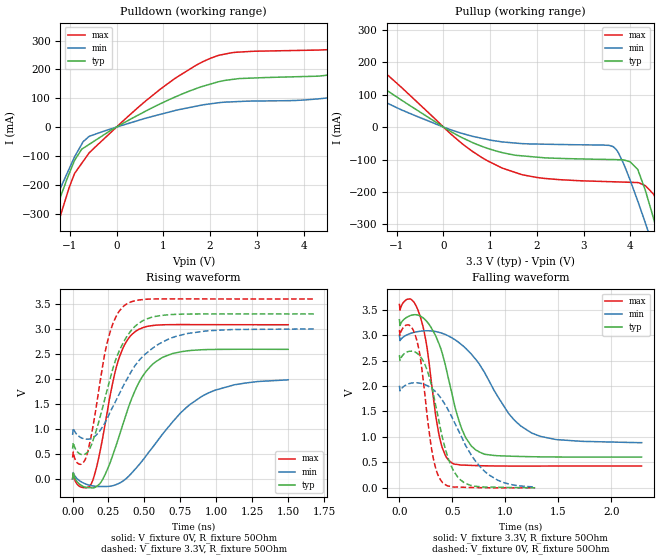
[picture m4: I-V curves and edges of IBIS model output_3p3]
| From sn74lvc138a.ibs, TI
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|   output_3p3 Model
[Model]   output_3p3
Model_type   Output
Polarity   Non-Inverting
Vmeas = 1.65
Vref = 1.65
Cref = 2pF
Rref = 50
|   typ   min   max
|   (nom PVT)   (fast PVT)   (slow PVT)
|C_comp from frequency sweep method (F=5MHz)
|C_comp   6.810e-12   6.693e-12   8.623e-12
|ON state : BUFFER OUTPUT TURNED HIGH
|C_comp   6.810e-12   6.693e-12   8.623e-12
|OFF state: BUFFER OUTPUT TURNED LOW
|C_comp   6.538e-12   6.289e-12   6.590e-12
|C_comp from LC tank measurement(L=1nH)
|Resonant Frequency(Hz)   2.010e+09   2.070e+09   1.960e+09
C_comp   6.276e-12   5.917e-12   6.600e-12
|ON state : BUFFER OUTPUT TURNED HIGH
|Resonant Frequency(Hz)   2.010e+09   2.070e+09   1.960e+09
|C_comp   6.276e-12   5.917e-12   6.600e-12
|OFF state: BUFFER OUTPUT TURNED LOW
|Resonant Frequency(Hz)   2.260e+09   2.290e+09   2.140e+09
|C_comp   4.964e-12   4.835e-12   5.537e-12
| Where nom  PVT is Nominal Process, 3.3V, 27C
|   Fast PVT is Strong Process,  3.6V, -40C
|   Slow PVT is Weak Process,   3V, 125C
[Voltage Range]   3.3   3   3.6
|Ambient Temperature   25   85   -40
|Junction Temperature
[Temperature Range]   27   125   -40
[Pullup Reference]   3.3   3   3.6
[Pulldown Reference]   0   0   0
[Power Clamp Reference]   3.3   3   3.6
[GND Clamp Reference]   0   0   0
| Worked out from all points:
|   slope of the pulldown table from 0 to 0.495 V, typ, clamps not added: 11.2 ohm
|   slope of the pullup table from 0 to 0.495 V, typ, clamps not added: 12.6 ohm
|   falling waveform, V_fixture 3.3V, R_fixture 50Ohm: 20-80 % time 206ps typ, 396ps min, 129ps max; typ from 3.3 V to 0.604 V
|   rising waveform, V_fixture 0V, R_fixture 50Ohm: 20-80 % time 207ps typ, 371ps min, 134ps max; typ from 0 V to 2.59 V
|   rising waveform, V_fixture 3.3V, R_fixture 50Ohm: 20-80 % time 177ps typ, 283ps min, 121ps max; typ from 0.605 V to 3.3 V
|   falling waveform, V_fixture 0V, R_fixture 50Ohm: 20-80 % time 177ps typ, 323ps min, 114ps max; typ from 2.61 V to 0.001 V
[Pulldown]
|   Voltage   I(typ)   I(min)   I(max)
-3.3V     -1.387A    -1.148A    -1.732A
-1.689V   -475.7mA   -405.4mA   -579.7mA
-1.308V   -291.1mA   -250.7mA   -366.8mA
-897.6mV  -115.5mA   -103mA     -161.1mA
-745.8mV  -76.85mA   -59.62mA   -126.1mA
-591mV    -60.58mA   -32.91mA   -90.57mA
939.6mV   81.03mA    44.25mA    131.8mA
2.012V    149.3mA    80.72mA    239mA
2.542V    166.6mA    88.11mA    259.4mA
4.95V     191.9mA    111mA      279.8mA
6V        240.9mA    146mA      341mA
6.6V      273.7mA    165.9mA    382.6mA
[Pullup]
|   Voltage   I(typ)   I(min)   I(max)
-3.3V     312.5mA    216.6mA    431.8mA
-3V       283.8mA    196.2mA    393.1mA
-897.6mV  83.18mA    52.99mA    122.3mA
392.4mV   -32.21mA   -19.31mA   -50.19mA
1.246V    -78.24mA   -45.48mA   -125.5mA
3.63V     -100.1mA   -60.21mA   -168.6mA
4.158V    -130.7mA   -228.1mA   -171.1mA
4.331V    -200.3mA   -299.9mA   -182mA
4.468V    -267.5mA   -358.7mA   -202.7mA
4.687V    -384.2mA   -456.2mA   -293.7mA
4.848V    -470.4mA   -528.2mA   -403mA
6.6V      -1.488A    -1.345A    -1.68A
[Ramp]
R_load = 50
|   typ   min   max
dV/dt_r   1.55471/2.06702e-10   1.19608/3.73506e-10   1.85065/1.33968e-10
dV/dt_f   1.61692/2.05325e-10   1.27163/3.97542e-10   1.90305/1.28863e-10
[Falling Waveform]
V_fixture = 3.3V
V_fixture_min = 3V
V_fixture_max = 3.6V
R_fixture = 50Ohm
|   Time   V(typ)   V(min)   V(max)
0s        3.3V       3V         3.6V
105ps     3.384V     3.032V     3.707V
190ps     3.381V     3.073V     3.402V
255ps     3.274V     3.084V     2.822V
380ps     2.792V     3.049V     977.3mV
495ps     1.853V     2.945V     489.2mV
590ps     1.148V     2.804V     446.4mV
720ps     743.4mV    2.522V     436.8mV
1.24ns    610.7mV    1.086V     427.1mV
2.285ns   604.3mV    886.8mV    428.3mV
[Rising Waveform]
V_fixture = 0V
V_fixture_min = 0V
V_fixture_max = 0V
R_fixture = 50Ohm
|   Time   V(typ)   V(min)   V(max)
0s        140.8pV    11.06nV    81.11pV
5ps       119.8mV    127.3mV    106.4mV
50ps      -107.5mV   -38.71mV   -151.7mV
130ps     -177.4mV   -133.6mV   -100.1mV
210ps     -6.53mV    -151.9mV   830.3mV
315ps     774.7mV    -98.27mV   2.34V
440ps     1.801V     209.7mV    2.956V
620ps     2.421V     873.8mV    3.082V
900ps     2.584V     1.652V     3.087V
1.5ns     2.593V     1.982V     3.084V
[Rising Waveform]
V_fixture = 3.3V
V_fixture_min = 3V
V_fixture_max = 3.6V
R_fixture = 50Ohm
|   Time   V(typ)   V(min)   V(max)
0s        605.1mV    880.6mV    428.2mV
55ps      496.5mV    831.9mV    292.3mV
95ps      512.4mV    796mV      435.8mV
155ps     880.8mV    853.5mV    1.273V
240ps     1.774V     1.203V     2.715V
300ps     2.382V     1.556V     3.232V
365ps     2.791V     1.925V     3.478V
495ps     3.174V     2.469V     3.59V
725ps     3.293V     2.856V     3.602V
1.685ns   3.3V       3V         3.6V
[Falling Waveform]
V_fixture = 0V
V_fixture_min = 0V
V_fixture_max = 0V
R_fixture = 50Ohm
|   Time   V(typ)   V(min)   V(max)
0s        2.607V     2.003V     3.102V
95ps      2.682V     2.048V     3.191V
160ps     2.652V     2.063V     2.925V
205ps     2.555V     2.049V     2.44V
315ps     1.895V     1.934V     627.8mV
405ps     990.6mV    1.719V     107.7mV
500ps     376.6mV    1.368V     18.43mV
615ps     95.55mV    873.2mV    10.05mV
845ps     15.26mV    252.7mV    735.3uV
1.28ns    990.1uV    15.75mV    -540.3uV
